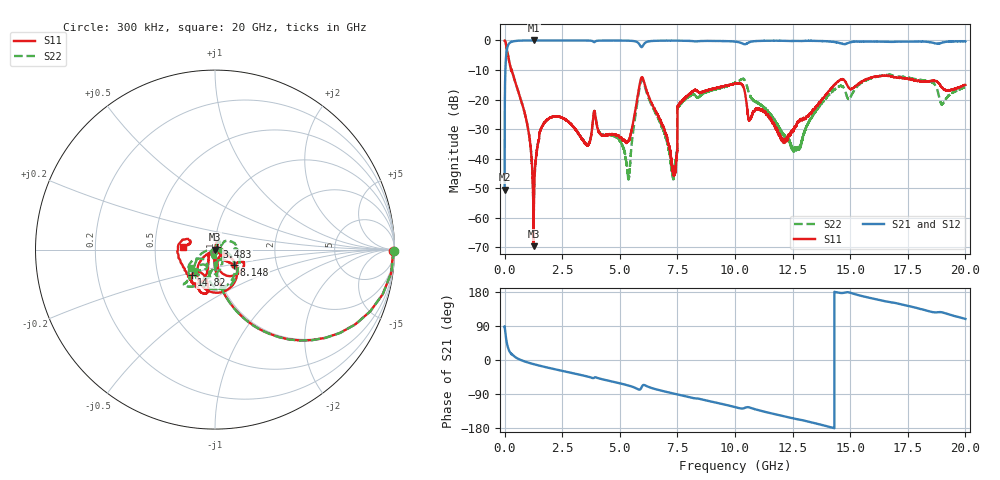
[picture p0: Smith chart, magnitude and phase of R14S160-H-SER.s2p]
!{R14S160}
!Johanson Technology Inc.
!www.johansontechnology.com
!Test Board Conditions:
!Substrate Type  RO4350B
!Substrate Thickness  20 mil
!Substrate Dk  3.66
!TL Type: GCPW
!TL Trace Width  36 mil
!TL Gap  12 mil
!Electrode orientation  Horizontal
!DUT TOPOLOGY	SERIES
!Mounting Pad LxW  26x36 mil
! Created Wed Nov 25 17:33:21 2020
! 2 Port Network Data from SP1.SP block
! freq  magS11  angS11  magS21  angS21  magS12  angS12  magS22  angS22
# khz S ma R 50
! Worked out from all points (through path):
!   20001 points, 300 kHz to 20 GHz, reference 50 ohm
!   highest |S21| = 0.00 dB at 1.283 GHz (marker M1); lowest = -50.5 dB at 300 kHz (marker M2)
!   group delay of S21, straight-line fit = 35.7 ps
!   lowest |S11| = -69.6 dB at 1.262 GHz (marker M3), VSWR 1.00, Z = 50 + j0.0289 ohm
!   |S11| at or under -10 dB: 285.2 MHz to 300 MHz (14.76 MHz wide, 5.05 % of centre); 307.6 MHz to end of sweep
!   |S22| runs from -61.9 to 0.0 dB; largest |S21 - S12| = 0.017
!   S11 on the Smith chart (normalised r, x): 300 kHz: open; 3.483 GHz: 1.02, +0.03; 8.148 GHz: 1.22, -0.21; 14.82 GHz: 0.74, -0.22; 20 GHz: 0.70, +0.02
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300  0.993 -0.4  0.002997 88.6  0.002972 90.4  0.998 -0.3
165300  0.5111 -60.5  0.8565 29.4  0.8573 29.3  0.5133 -60.5
959300  0.04233 -95.4  0.9983 -5.6  0.9982 -5.6  0.04265 -95.2
1262300  0.000332 119.3  0.9993 -10.9  0.9989 -10.9  0.001241 -6.1
1283300  0.002669 93.1  1 -11.3  0.999 -11.3  0.002822 58.9
1849300  0.04573 74.8  0.9976 -19.8  0.9984 -19.8  0.0457 64.8
3334300  0.02225 56.5  0.9974 -39.8  0.9977 -39.9  0.02227 32.4
3483300  0.01808 52.3  0.9971 -42.0  0.9973 -41.9  0.0184 27.4
3919300  0.06048 -76.4  0.948 -45.7  0.948 -45.7  0.06107 -79.3
5371300  0.0198 -65.1  0.9904 -67.3  0.9907 -67.3  0.005181 104.4
5962300  0.2408 -85.6  0.774 -70.0  0.7734 -70.0  0.2217 -90.0
6667300  0.05295 -148.7  0.9886 -78.9  0.9882 -78.9  0.04773 -172.5
7353300  0.005604 -65.7  0.9943 -88.7  0.9934 -88.8  0.005846 -68.5
7600300  0.08614 -46.4  0.9895 -92.2  0.9894 -92.2  0.08039 36.9
8148300  0.1361 -38.9  0.9751 -99.9  0.975 -99.9  0.1206 10.3
1.00003e7  0.1856 -29.7  0.955 -124.3  0.9558 -124.3  0.1923 -53.4
1.06433e7  0.04604 -39.9  0.9385 -125.6  0.9408 -125.6  0.1192 -98.8
1.25583e7  0.03158 -131.8  0.9806 -154.4  0.9805 -154.4  0.01445 -54.3
1.33343e7  0.06118 -125.3  0.9844 -164.9  0.9858 -164.9  0.04974 -38.0
1.48203e7  0.1925 -132.8  0.8765 178.6  0.8764 178.5  0.1261 -134.3
1.66673e7  0.2512 -107.5  0.9521 153.3  0.9446 153.2  0.2636 -129.7
2e7  0.1781 175.1  0.9662 108.4  0.9655 108.5  0.1652 -143.1
